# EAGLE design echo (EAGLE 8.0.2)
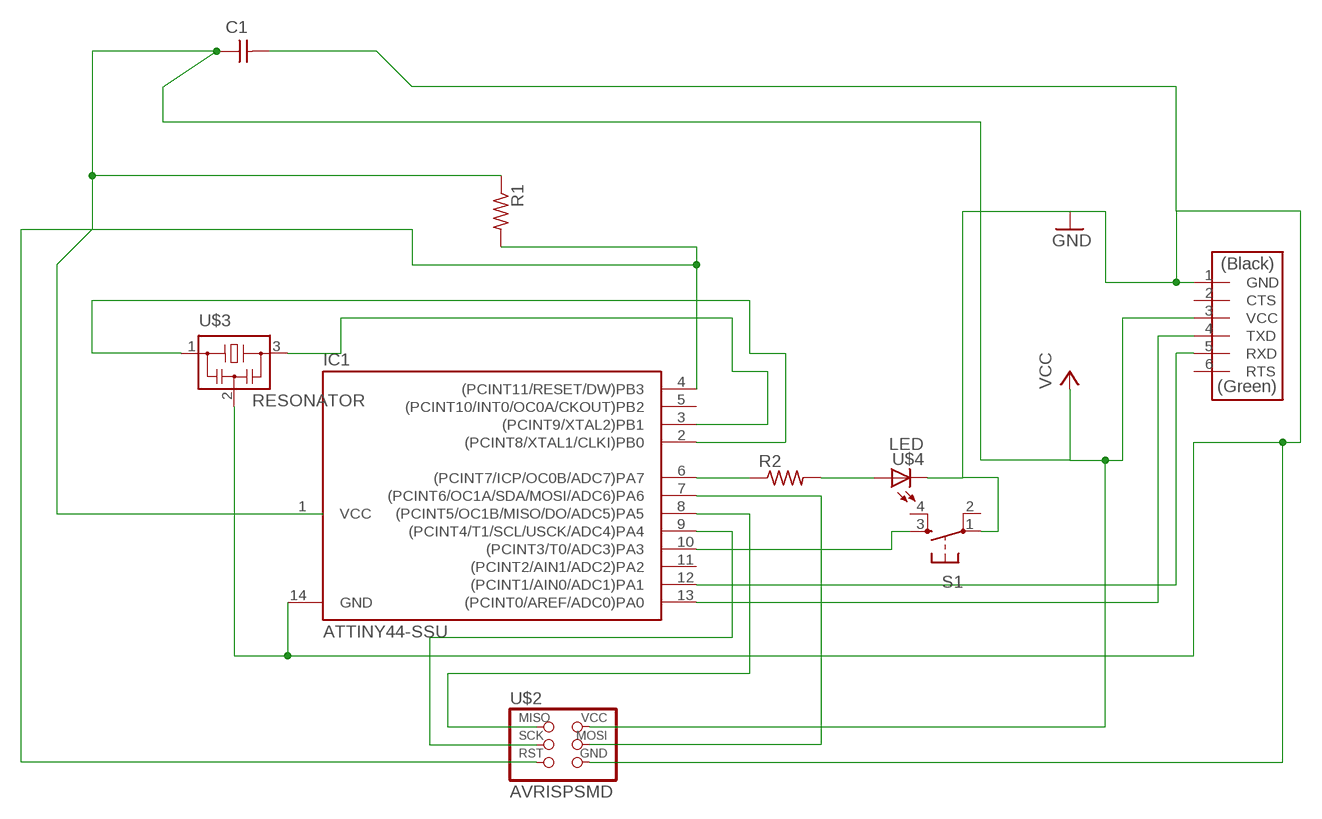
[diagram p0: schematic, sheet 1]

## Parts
C1  CAP-UNPOLARIZEDFAB  [C1206FAB]
IC1  ATTINY44-SSU  [SOIC14]
R1  RES-US1206FAB  [R1206FAB]
R2  RES-US1206FAB  [R1206FAB]
S1  6MM_SWITCH6MM_SWITCH  [6MM_SWITCH]
U$1  FTDI-SMD-HEADER  [1X06SMD]
U$2  AVRISPSMD  [2X03SMD]
U$3  RESONATOR  [EFOBM]
U$4  LED  [LED1206]

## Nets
GND: C1.2 IC1.14(GND) S1.1(P) U$1.1(GND) U$2.6(GND) U$3.2 U$4.2(C)
N$1: IC1.2((PCINT8/XTAL1/CLKI)PB0) U$3.1
N$2: IC1.3((PCINT9/XTAL2)PB1) U$3.3
N$4: IC1.4((PCINT11/RESET/DW)PB3) R1.2 U$2.5(RST)
N$5: IC1.7((PCINT6/OC1A/SDA/MOSI/ADC6)PA6) U$2.4(MOSI)
N$6: IC1.8((PCINT5/OC1B/MISO/DO/ADC5)PA5) U$2.1(MISO)
N$7: IC1.9((PCINT4/T1/SCL/USCK/ADC4)PA4) U$2.3(SCK)
N$8: IC1.12((PCINT1/AIN0/ADC1)PA1) U$1.5(RXD)
N$9: IC1.13((PCINT0/AREF/ADC0)PA0) U$1.4(TXD)
N$10: IC1.6((PCINT7/ICP/OC0B/ADC7)PA7) R2.1
N$11: R2.2 U$4.1(A)
N$12: IC1.10((PCINT3/T0/ADC3)PA3) S1.3(S)
VCC: C1.1 IC1.1(VCC) R1.1 U$1.3(VCC) U$2.2(VCC)
Unconnected: IC1.5((PCINT10/INT0/OC0A/CKOUT)PB2) IC1.11((PCINT2/AIN1/ADC2)PA2) S1.2(P1) S1.4(S1) U$1.2(CTS) U$1.6(RTS)

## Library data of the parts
C1 = fab:CAP-UNPOLARIZED
IC1 = fab:ATTINY44
R1 R2 = fab:RES-US: Resistor (US Symbol)
S1 = fab:6MM_SWITCH: OMRON SWITCH
U$1 = fab:FTDI-SMD-HEADER
U$2 = fab:AVRISP
U$3 = fab:RESONATOR
U$4 = fab:LED: LED

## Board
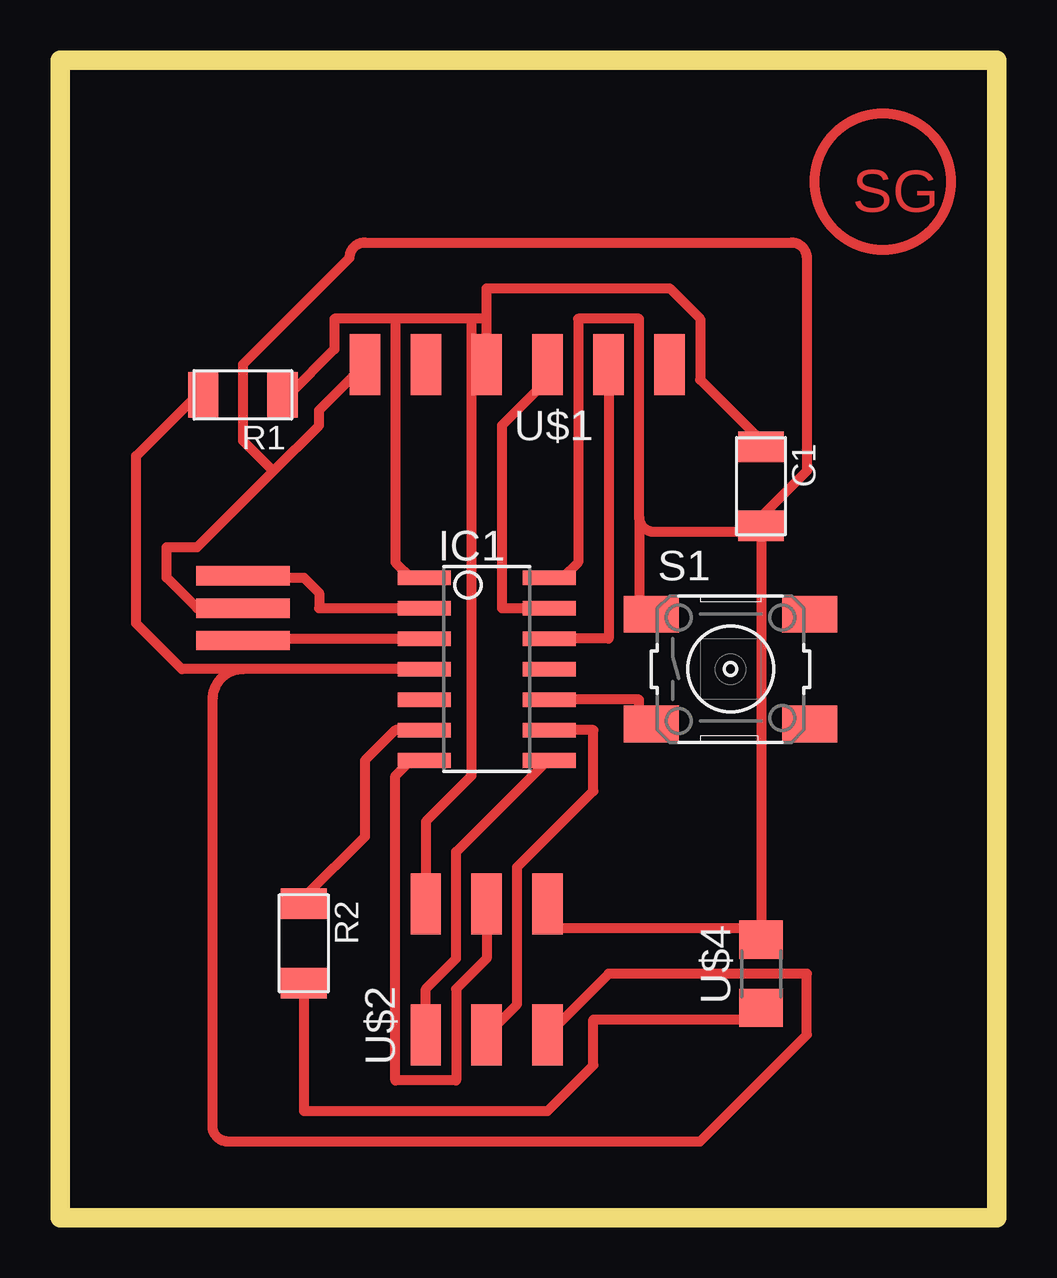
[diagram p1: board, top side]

Size 39.04 x 48.25 mm. Coordinates in mm from the lower left corner, seen from the top.
Outline: 0,0 39.04,0 39.04,48.25 0,48.25 0,0
Copper layers (1*16): Top 0.035mm / dielectric 1.5mm / Bottom 0.035mm
Design rules "default *": minimum track width 16mil, minimum drill 24mil, track to track 16mil, track to pad 16mil, pad to pad 16mil, via to via 16mil, smd to smd 8mil, copper to edge 40mil, drill to drill 8mil, minimum pad ring 10mil, minimum via ring 8mil, stop-mask expansion 4mil, vias tented up to drill 0mil, thermal gap 10mil

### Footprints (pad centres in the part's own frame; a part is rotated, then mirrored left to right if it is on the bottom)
C1206FAB = smd 1.27 x 1.905: 1 -1.651,0; 2 1.651,0
SOIC14 = smd 0.61 x 2.21: 1 -3.81,-2.603; 2 -2.54,-2.603; 3 -1.27,-2.603; 4 0,-2.603; 5 1.27,-2.603; 6 2.54,-2.603; 7 3.81,-2.603; 8 3.81,2.603; 9 2.54,2.603; 10 1.27,2.603; 11 0,2.603; 12 -1.27,2.603; 13 -2.54,2.603; 14 -3.81,2.603
R1206FAB = smd 1.27 x 1.905: 1 -1.651,0; 2 1.651,0
6MM_SWITCH = smd 2.286 x 1.524: 1 -3.302,2.286; 2 3.302,2.286; 3 -3.302,-2.286; 4 3.302,-2.286
1X06SMD = smd 2.54 x 1.27: 1 0,6.35; 2 0,3.81; 3 0,1.27; 4 0,-1.27; 5 0,-3.81; 6 0,-6.35
2X03SMD = smd 2.54 x 1.27: 1 -2.54,2.54; 2 2.92,2.54; 3 -2.54,0; 4 2.92,0; 5 -2.54,-2.54; 6 2.92,-2.54
EFOBM = smd 0.8 x 3.9: 1 -1.35,0; 2 0,0; 3 1.35,0
LED1206 = smd 1.6 x 1.803: 1 -1.422,0; 2 1.422,0

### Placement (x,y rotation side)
C1  29.21,30.48 270 top
IC1  17.78,22.86 270 top
R1  7.62,34.29 180 top
R2  10.16,11.43 270 top
S1  27.94,22.86 0 top
U$1  19.05,35.56 90 top
U$2  17.78,10.16 90 top
U$3  7.62,25.4 270 top
U$4  29.21,10.16 90 top

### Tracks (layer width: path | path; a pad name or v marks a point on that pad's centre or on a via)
GND
  Top 0.406: U$1.1 10.79,33.66 10.79,33.02 8.89,31.12 | 8.89,31.12 5.71,27.94 4.45,27.94 4.45,26.67 5.71,25.4 U$3.2 | 29.21,12.07 20.32,12.07 U$2.6 | 29.21,28.58 24.76,28.58 arc-90 24.13,29.21 | 24.76,25.4 S1.1 24.13,25.4 24.13,29.21 | 24.13,29.21 24.13,37.47 21.59,37.47 21.59,27.3 20.95,26.67 IC1.14 | 29.21,28.58 29.21,12.07 | 29.21,12.07 U$4.2 | 29.21,28.58 C1.2 29.21,29.21 31.12,31.12 31.12,40.01 arc90 30.48,40.64 12.7,40.64 arc90 12.06,40.01 7.62,35.56 7.62,32.38 8.89,31.12
N$1
  Top 0.406: IC1.2 10.79,25.4 10.79,26.04 10.16,26.67 7.62,26.67 U$3.1
N$2
  Top 0.406: IC1.3 7.62,24.13 U$3.3
N$4
  Top 0.406: IC1.4 7.62,22.86 | 7.62,22.86 5.08,22.86 3.17,24.77 3.17,31.75 5.71,34.29 R1.2 | U$2.5 22.86,10.16 31.12,10.16 31.12,7.62 26.67,3.18 6.98,3.18 arc-90 6.35,3.81 6.35,21.59 arc-90 7.62,22.86
N$5
  Top 0.406: U$2.4 17.78,10.8 16.51,9.52 16.51,5.71 13.97,5.71 13.97,18.41 14.6,19.05 IC1.7
N$6
  Top 0.406: U$2.1 15.24,9.52 16.51,10.8 16.51,15.24 20.32,19.05 IC1.8
N$7
  Top 0.406: IC1.9 22.22,20.32 22.22,17.78 19.05,14.61 19.05,8.89 U$2.3
N$8
  Top 0.406: IC1.12 22.86,24.13 U$1.5
N$9
  Top 0.406: IC1.13 18.41,25.4 18.41,33.02 20.32,34.93 U$1.4
N$10
  Top 0.406: IC1.6 13.97,20.32 12.7,19.05 12.7,15.88 10.16,13.34 R2.1
N$11
  Top 0.406: R2.2 10.16,4.45 20.32,4.45 22.22,6.35 22.22,8.26 29.21,8.26 U$4.1
N$12
  Top 0.406: IC1.10 24.13,21.59 24.13,20.95 S1.3
VCC
  Top 0.406: U$1.3 17.78,37.47 | 17.78,37.47 17.78,38.74 25.4,38.74 26.67,37.47 26.67,34.93 29.21,32.38 C1.1 | 17.78,37.47 17.14,37.47 | 17.14,37.47 13.97,37.47 | 13.97,37.47 11.43,37.47 11.43,36.2 9.52,34.29 R1.1 | 13.97,37.47 13.97,27.3 14.6,26.67 IC1.1 | U$2.2 15.24,16.51 17.14,18.41 17.14,37.47
(copper drawn outside any net)
  shapes: Top circle x1

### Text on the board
Top: SG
